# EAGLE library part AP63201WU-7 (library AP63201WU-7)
VIN 3.8V to 32V 2A Continuous Output Current 0.8V +/- 1% Reference Voltage 22A Ultralow Quiescent Current Switching Frequency o 500kHz: AP63200 and AP63201 o 1.1MHz: AP63203 and AP63205 Pulse Width Modulation (PWM) Regardless of Output Load o AP63201 Supports Pulse Frequency Modulation (PFM) o AP63200, AP63203, and AP63205 o Up to 80% Efficiency at 1mA Light Load o Up to 88% Efficiency at 5mA Light Load Fixed Output Voltage o 3.3V: AP63203 o 5.0V: AP63205 Proprietary Gate Dr Source: Datasheet
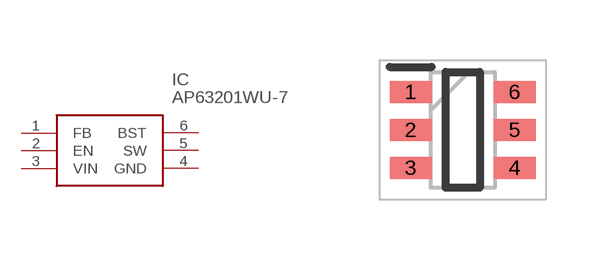
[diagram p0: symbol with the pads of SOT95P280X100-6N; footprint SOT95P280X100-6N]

Designator prefix IC

## AP63201WU-7 (Arrow_Part_Number: AP63201WU-7; Arrow_Price-Stock: https://www.arrow.com/en/products/ap63201wu-7/diodes-incorporated?region=nac; Description: VIN 3.8V to 32V 2A Continuous Output Current 0.8V +/- 1% Reference Voltage 22A Ultralow Quiescent Current Switching Frequency o 500kHz: AP63200 and AP63201 o 1.1MHz: AP63203 and AP63205 Pulse Width Modulation (PWM) Regardless of Output Load o AP63201 Supports Pulse Frequency Modulation (PFM) o AP63200, AP63203, and AP63205 o Up to 80% Efficiency at 1mA Light Load o Up to 88% Efficiency at 5mA Light Load Fixed Output Voltage o 3.3V: AP63203 o 5.0V: AP63205 Proprietary Gate Dr; Height: 1mm; Manufacturer_Name: Diodes Incorporated; Manufacturer_Part_Number: AP63201WU-7; Mouser_Part_Number: 621-AP63201WU-7; Mouser_Price-Stock: https://www.mouser.co.uk/ProductDetail/Diodes-Incorporated/AP63201WU-7?qs=u16ybLDytRaVD%252BU3eG30NA%3D%3D)  [SOT95P280X100-6N]
1  FB
2  EN
3  VIN
4  GND
5  SW
6  BST

## Footprint SOT95P280X100-6N (pad centres in mm)
TSOT26 (Standard)_2024
smd 1.05 x 0.55: 1 -1.3,0.95; 2 -1.3,0; 3 -1.3,-0.95; 4 1.3,-0.95; 5 1.3,0; 6 1.3,0.95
